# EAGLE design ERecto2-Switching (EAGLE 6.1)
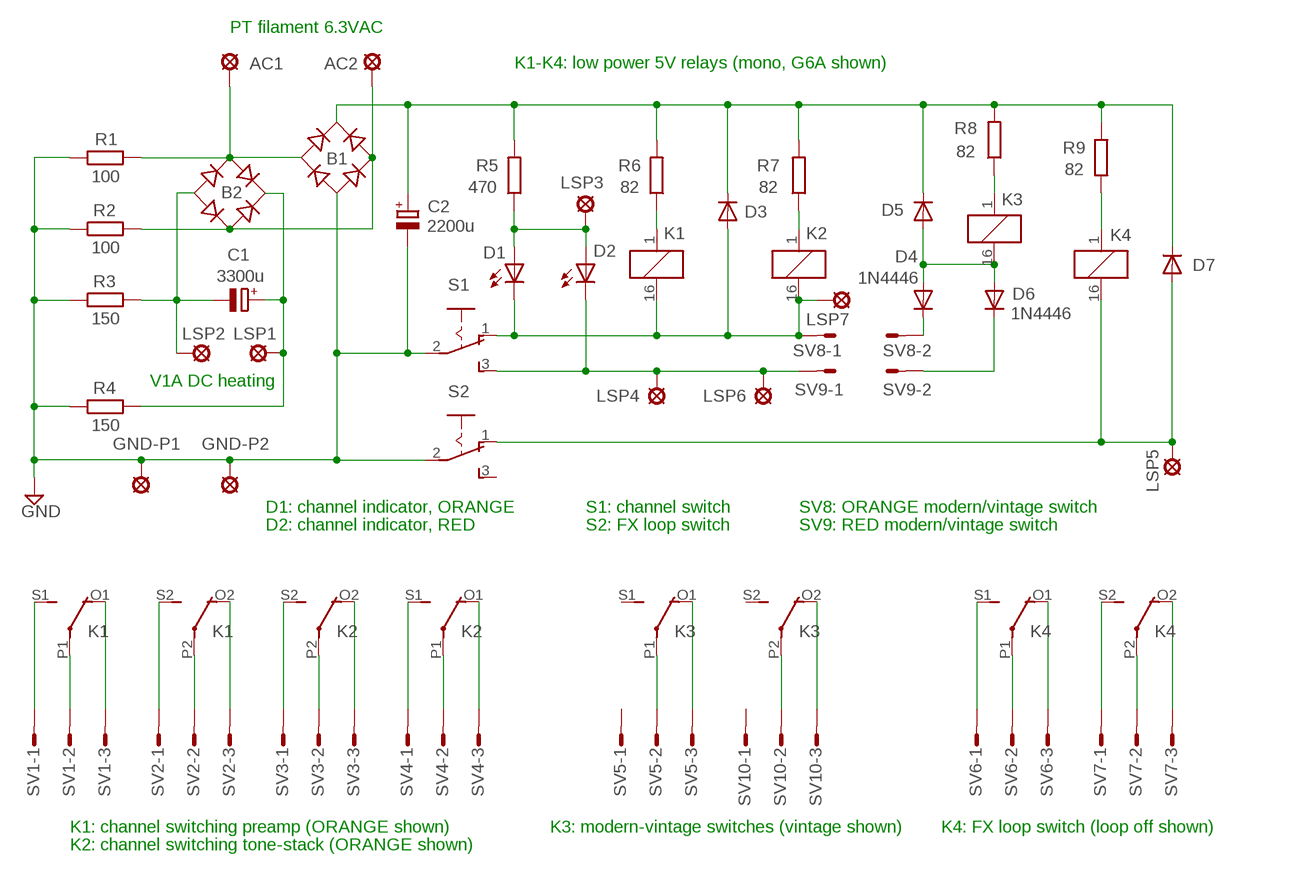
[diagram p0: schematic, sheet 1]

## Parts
AC1  SE13  [SE13]
AC2  SE13  [SE13]
B1  RECTIFIER-RB1A  [RB1A]
B2  RECTIFIER-RB1A  [RB1A]
C1  3300u  CPOL-EUE5-13  [E5-13]
C2  2200u  CPOL-EUE5-13  [E5-13]
D1  LED5MM  [LED5MM]
D2  LED5MM  [LED5MM]
D3  1N4148DO35-10  [DO35-10]
D4  1N4446  [DO35-10]
D5  1N4148DO35-10  [DO35-10]
D6  1N4446  [DO35-10]
D7  1N4148DO35-10  [DO35-10]
GND-P1  SE13  [SE13]
GND-P2  SE13  [SE13]
K1  G6A-234P  [G6A-234P]
K2  G6A-234P  [G6A-234P]
K3  G6A-234P  [G6A-234P]
K4  G6A-234P  [G6A-234P]
LSP1  SE13  [SE13]
LSP2  SE13  [SE13]
LSP3  SE13  [SE13]
LSP4  SE13  [SE13]
LSP5  SE13  [SE13]
LSP6  SE13  [SE13]
LSP7  SE13  [SE13]
R1  100  R-EU_0207/10  [0207/10]
R2  100  R-EU_0207/10  [0207/10]
R3  150  R-EU_0207/10  [0207/10]
R4  150  R-EU_0207/10  [0207/10]
R5  470  R-EU_0207/10  [0207/10]
R6  82  R-EU_0207/10  [0207/10]
R7  82  R-EU_0207/10  [0207/10]
R8  82  R-EU_0207/10  [0207/10]
R9  82  R-EU_0207/10  [0207/10]
S1  255SB  [255SB]
S2  255SB  [255SB]
SV1  S03P  [S03P]
SV2  S03P  [S03P]
SV3  S03P  [S03P]
SV4  S03P  [S03P]
SV5  S03P  [S03P]
SV6  S03P  [S03P]
SV7  S03P  [S03P]
SV8  S02P  [S02P]
SV9  S02P  [S02P]
SV10  S03P  [S03P]

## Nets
GND: B1.- C2.- GND-P1.MP GND-P2.MP R1.1 R2.1 R3.1 R4.1 S1.2(P) S2.2(P)
N$1: B1.+ C2.+ D3.C D5.C D7.C R5.2 R6.2 R7.2 R8.2 R9.2
N$2: K1.1 R6.1
N$3: AC1.MP B1.AC1 B2.AC1 R1.2
N$4: AC2.MP B1.AC2 B2.AC2 R2.2
N$5: D1.K(C) D3.A K1.16 K2.16 LSP7.MP S1.1(O) SV8.1
N$6: D7.A K4.16 LSP5.MP S2.1(O)
N$7: K1.S1(2:S) SV1.1
N$8: K1.P1(2:P) SV1.2
N$9: K1.O1(2:O) SV1.3
N$10: K1.S2(3:S) SV2.1
N$11: K1.P2(3:P) SV2.2
N$12: K1.O2(3:O) SV2.3
N$13: K2.S2(3:S) SV3.1
N$14: K2.P2(3:P) SV3.2
N$15: K2.O2(3:O) SV3.3
N$16: K2.S1(2:S) SV4.1
N$17: K2.P1(2:P) SV4.2
N$18: K2.O1(2:O) SV4.3
N$19: K3.P2(3:P) SV10.2
N$20: K3.P1(2:P) SV5.2
N$21: K3.O1(2:O) SV5.3
N$22: K4.S1(2:S) SV6.1
N$23: K4.P1(2:P) SV6.2
N$24: K4.O1(2:O) SV6.3
N$25: K4.S2(3:S) SV7.1
N$26: K4.P2(3:P) SV7.2
N$27: K4.O2(3:O) SV7.3
N$28: B2.- C1.- LSP2.MP R3.2
N$29: B2.+ C1.+ LSP1.MP R4.2
N$30: K2.1 R7.1
N$31: K3.1 R8.1
N$32: D4.C SV8.2
N$33: D4.A D5.A D6.A K3.16
N$34: D2.K(C) LSP4.MP LSP6.MP S1.3(S) SV9.1
N$35: K4.1 R9.1
N$36: D6.C SV9.2
N$37: K3.O2(3:O) SV10.3
N$41: D1.A D2.A LSP3.MP R5.1
Unconnected: K3.S1(2:S) K3.S2(3:S) S2.3(S) SV5.1 SV10.1

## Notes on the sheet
- PT filament 6.3VAC
- K1-K4: low power 5V relays (mono, G6A shown)
- V1A DC heating
- D1: channel indicator, ORANGE | S1: channel switch | SV8: ORANGE modern/vintage switch
- D2: channel indicator, RED | S2: FX loop switch | SV9: RED modern/vintage switch
- K1: channel switching preamp (ORANGE shown) | K3: modern-vintage switches (vintage shown) | K4: FX loop switch (loop off shown)
- K2: channel switching tone-stack (ORANGE shown)

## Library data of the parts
AC1 AC2 GND-P1 GND-P2 LSP1-LSP7 = solpad:SE13: SOLDER PAD
B1 B2 = rectifier:RECTIFIER-: Rectifier
C1 C2 = resistor:CPOL-EU: POLARIZED CAPACITOR, European symbol
D1 D2 = led:LED: LED
D3 D5 D7 = diode:1N4148: DIODE
D4 D6 = diode:1N4446: DIODE
K1-K4 = relay:G6A-234P: RELAY 2 x switch, 0.3 A/125 V AC, 1 A/30 V DC, Omron; OC_FARNELL: unknown; OC_NEWARK: unknown
R1-R9 = rcl:R-EU_: RESISTOR, European symbol
S1 S2 = switch:255SB: SLIDING SWITCH Distributor Buerklin, 11G810
SV1-SV7 SV10 = con-amp-mt:S03P: AMP MT CONNECTOR; OC_FARNELL: unknown; OC_NEWARK: unknown
SV8 SV9 = con-amp-mt:S02P: AMP MT CONNECTOR; OC_FARNELL: unknown; OC_NEWARK: unknown

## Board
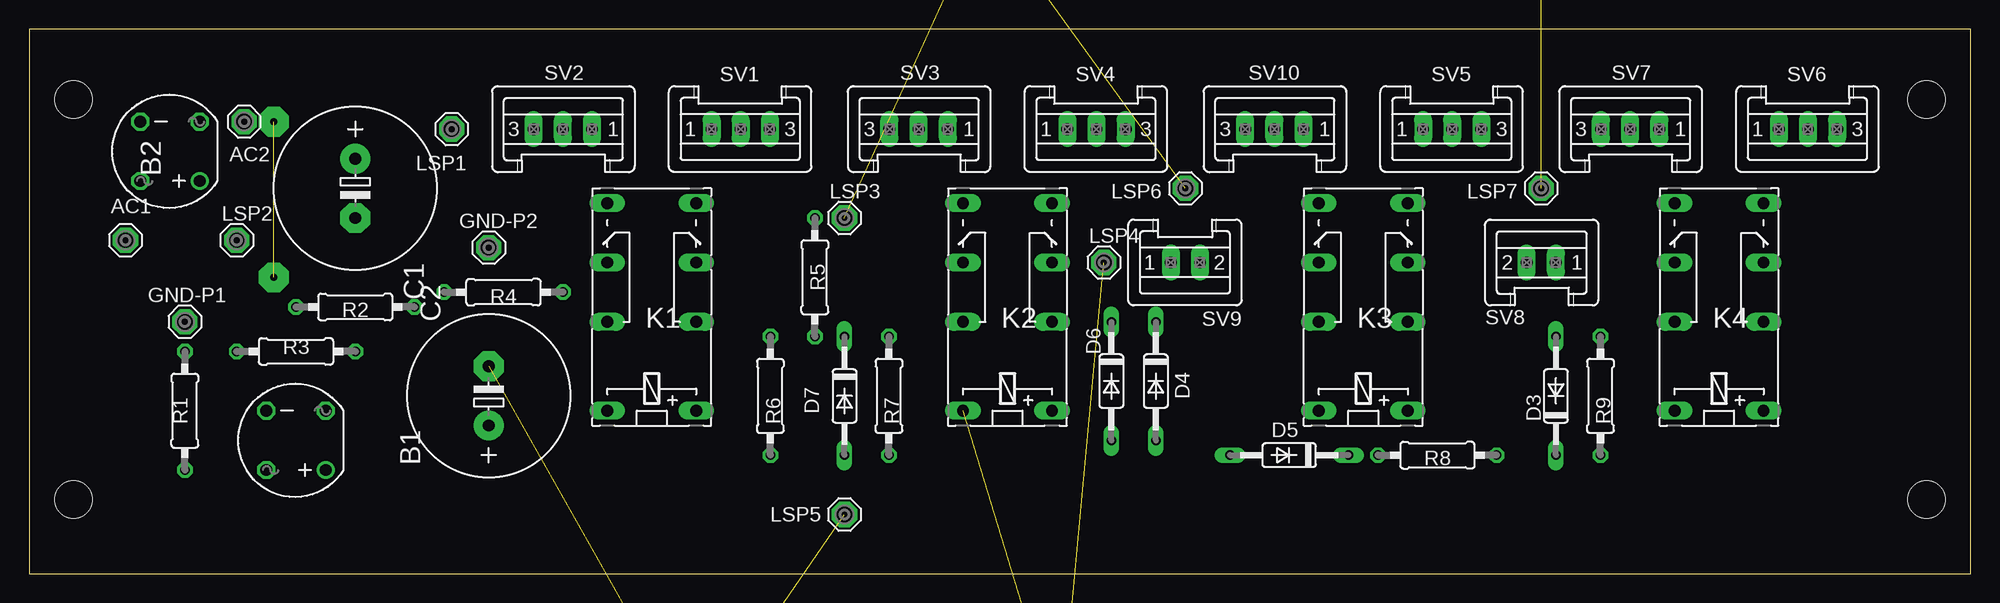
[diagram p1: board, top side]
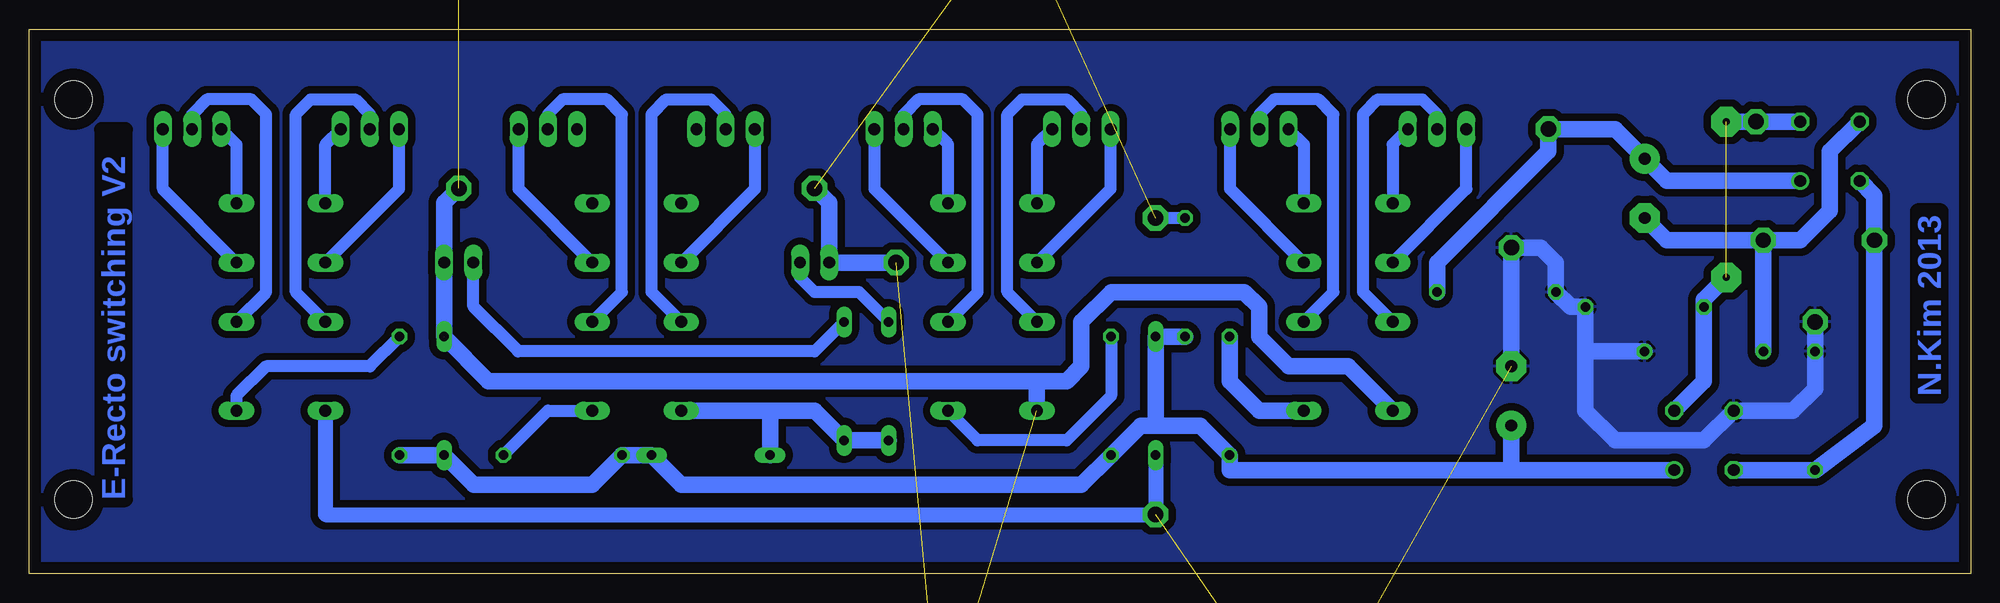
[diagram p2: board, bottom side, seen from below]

Size 166.35 x 46.66 mm. Coordinates in mm from the lower left corner, seen from the top.
Outline: 0,0 166.35,0 166.35,46.66 0,46.66 0,0
Copper layers (1*16): Top 0.035mm / dielectric 1.5mm / Bottom 0.035mm
Design rules: minimum track width 10mil, minimum drill 24mil, track to track 8mil, track to pad 8mil, pad to pad 8mil, via to via 8mil, smd to smd 8mil, copper to edge 40mil, drill to drill 8mil, minimum pad ring 10mil, minimum via ring 8mil, stop-mask expansion 4mil, vias tented up to drill 0mil, thermal gap 10mil
Holes 3.2 mm at 162.56,40.64 162.56,6.35 3.81,40.64 3.81,6.35

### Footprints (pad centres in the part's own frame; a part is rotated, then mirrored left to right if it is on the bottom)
SE13 = drill 1.321 pad 2.159 octagon: MP 0,0
RB1A = drill 1.016: + -2.54,2.54 | drill 1.016 octagon: - 2.54,-2.54; AC1 2.54,2.54; AC2 -2.54,-2.54
E5-13 = drill 1.016 pad 2.54: + -2.54,0 | drill 1.016 pad 2.54 octagon: - 2.54,0
LED5MM = drill 0.813 octagon: A -1.27,0; K 1.27,0
DO35-10 = drill 0.813 long: A 5.08,0; C -5.08,0
G6A-234P = drill 1.016 long: 1 -3.81,-3.81; 16 -3.81,3.81; O1 8.89,-3.81; O2 8.89,3.81; P1 3.81,-3.81; P2 3.81,3.81; S1 13.97,-3.81; S2 13.97,3.81
0207/10 = drill 0.813 octagon: 1 -5.08,0; 2 5.08,0
255SB = drill 1.118 long: 1 -3.81,0; 2 0,0; 3 3.81,0
S03P = drill 1.016 long: 1 2.5,0; 2 0,0; 3 -2.5,0
S02P = drill 1.016 long: 1 1.25,0; 2 -1.25,0

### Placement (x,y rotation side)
AC1  8.25,28.58 0 top
AC2  18.41,38.73 0 top
B1  22.86,11.43 180 top
B2  12.06,36.2 180 top
C1  27.94,33.02 270 top
C2  39.37,15.24 90 top
D1  not placed on the board
D2  not placed on the board
D3  130.81,15.24 90 top
D4  96.52,16.51 270 top
D5  107.95,10.16 180 top
D6  92.71,16.51 270 top
D7  69.85,15.24 270 top
GND-P1  13.34,21.59 0 top
GND-P2  39.37,27.94 0 top
K1  53.34,17.78 90 top
K2  83.82,17.78 90 top
K3  114.3,17.78 90 top
K4  144.78,17.78 90 top
LSP1  36.2,38.1 0 top
LSP2  17.78,28.58 0 top
LSP3  69.85,30.48 0 top
LSP4  92.07,26.67 0 top
LSP5  69.85,5.08 0 top
LSP6  99.06,33.02 0 top
LSP7  129.54,33.02 0 top
R1  13.34,13.97 270 top
R2  27.94,22.86 180 top
R3  22.86,19.05 180 top
R4  40.64,24.13 0 top
R5  67.31,25.4 270 top
R6  63.5,15.24 270 top
R7  73.66,15.24 270 top
R8  120.65,10.16 180 top
R9  134.62,15.24 270 top
S1  not placed on the board
S2  not placed on the board
SV1  60.96,38.1 180 top
SV2  45.72,38.1 0 top
SV3  76.2,38.1 0 top
SV4  91.44,38.1 180 top
SV5  121.92,38.1 180 top
SV6  152.4,38.1 180 top
SV7  137.16,38.1 0 top
SV8  129.54,26.67 0 top
SV9  99.06,26.67 180 top
SV10  106.68,38.1 0 top

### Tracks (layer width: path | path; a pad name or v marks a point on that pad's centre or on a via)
GND  (2 unrouted)
  Bottom 1.422: 33.02,19.05 R2.1 34.29,22.86 R4.1 35.56,26.67 36.83,27.94 GND-P2.MP C2.- | 33.02,19.05 33.02,13.97 30.48,11.43 22.86,11.43 B1.- 15.24,13.97 13.34,15.88 R1.1 GND-P1.MP | R3.1 33.02,19.05
  pour Bottom (isolate 0.635): 0,46.99 166.37,46.99 166.37,0 0,0
N$1
  Bottom 1.422: 69.85,12.7 66.04,12.7 R6.2 63.5,8.89 39.37,8.89 | 69.85,12.7 71.12,12.7 R7.2 76.2,7.62 110.49,7.62 D5.C R8.2 118.11,7.62 128.27,7.62 D3.C R9.2 | 69.85,12.7 D7.C R5.2 | B1.+ 39.37,8.89 | C2.+ 39.37,8.89
N$2
  Bottom 1.422: R6.1 63.5,16.51 60.96,13.97 K1.1
N$3
  Bottom 1.422: B1.AC1 R1.2 8.25,12.7 AC1.MP 8.25,32.38 B2.AC1
N$4  (1 unrouted)
  Bottom 1.422: B1.AC2 22.86,16.51 R2.2 22.86,23.49 20.95,25.4 | B2.AC2 AC2.MP 20.95,38.73
N$5  (3 unrouted)
  Bottom 1.422: 80.01,16.51 127,16.51 130.79,20.3 SV8.1 130.79,31.77 LSP7.MP | 80.01,16.51 77.47,16.51 76.2,17.78 76.2,21.59 73.66,24.13 62.23,24.13 60.96,22.86 60.96,20.32 58.42,17.78 53.34,17.78 K1.16 | K2.16 80.01,16.51
N$6  (1 unrouted)
  Bottom 1.27: D7.A LSP5.MP 140.97,5.08 K4.16
N$7
  Bottom 1.016: SV1.1 57.15,36.79 K1.S1
N$8
  Bottom 1.016: K1.P1 54.61,24.13 54.61,39.37 55.88,40.64 59.69,40.64 60.96,39.37 SV1.2
N$9
  Bottom 1.016: K1.O1 63.46,32.98 SV1.3
N$10
  Bottom 1.016: SV2.1 49.53,36.79 K1.S2
N$11
  Bottom 1.016: K1.P2 52.07,24.13 52.07,39.37 50.8,40.64 46.99,40.64 45.72,39.37 SV2.2
N$12
  Bottom 1.016: K1.O2 43.22,32.98 SV2.3
N$13
  Bottom 1.016: SV3.1 80.01,36.79 K2.S2
N$14
  Bottom 1.016: K2.P2 82.55,24.13 82.55,39.37 81.28,40.64 77.47,40.64 76.2,39.37 SV3.2
N$15
  Bottom 1.016: K2.O2 73.7,32.98 SV3.3
N$16
  Bottom 1.016: K2.S1 87.63,36.79 SV4.1
N$17
  Bottom 1.016: K2.P1 85.09,24.13 85.09,39.37 86.36,40.64 90.17,40.64 91.44,39.37 SV4.2
N$18
  Bottom 1.016: SV4.3 93.94,32.98 K2.O1
N$19
  Bottom 1.016: K3.P2 113.03,24.13 113.03,39.37 111.76,40.64 107.95,40.64 106.68,39.37 SV10.2
N$20
  Bottom 1.016: K3.P1 115.57,24.13 115.57,39.37 116.84,40.64 120.65,40.64 121.92,39.37 SV5.2
N$21
  Bottom 1.016: K3.O1 124.42,32.98 SV5.3
N$22
  Bottom 1.016: SV6.1 148.59,36.79 K4.S1
N$23
  Bottom 1.016: K4.P1 146.05,24.13 146.05,39.37 147.32,40.64 151.13,40.64 152.4,39.37 SV6.2
N$24
  Bottom 1.016: K4.O1 154.9,32.98 SV6.3
N$25
  Bottom 1.016: K4.S2 140.97,36.79 SV7.1
N$26
  Bottom 1.016: K4.P2 143.51,24.13 143.51,39.37 142.24,40.64 138.43,40.64 137.16,39.37 SV7.2
N$27
  Bottom 1.016: K4.O2 134.66,32.98 SV7.3
N$28
  Bottom 1.422: LSP2.MP R3.2 | B2.- 12.06,36.2 12.06,31.12 14.61,28.58 LSP2.MP | C1.- 26.03,28.58 LSP2.MP
N$29
  Bottom 1.422: B2.+ 26.03,33.66 C1.+ 30.48,38.1 LSP1.MP 36.2,36.2 45.72,26.67 R4.2
N$30
  Bottom 1.016: R7.1 73.66,15.24 77.47,11.43 85.09,11.43 K2.1
N$31
  Bottom 1.016: R8.1 121.92,13.97 K3.1
N$32
  Bottom 1.016: D4.C 99.06,19.05 124.46,19.05 128.29,22.88 SV8.2
N$33
  Bottom 1.422: D6.A D4.A 99.06,13.97 102.87,13.97 | K3.16 102.87,13.97 | D5.A 102.87,13.97
N$34  (2 unrouted)
  Bottom 1.422: LSP6.MP 97.81,31.77 SV9.1 LSP4.MP
N$35
  Bottom 1.016: R9.1 137.16,17.78 146.05,17.78 148.59,15.24 K4.1
N$36
  Bottom 1.016: D6.C 95.25,24.13 99.06,24.13 100.31,25.38 SV9.2
N$37
  Bottom 1.016: SV10.3 104.18,32.98 K3.O2
N$38  (via drill 0.6 pad 2.54)
  other vias: 20.95,38.73
N$39  (via drill 0.6 pad 2.54)
  other vias: 20.95,25.4
N$41  (2 unrouted)
  Bottom 1.016: R5.1 LSP3.MP

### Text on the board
Bottom: N.Kim 2013 | E-Recto switching V2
